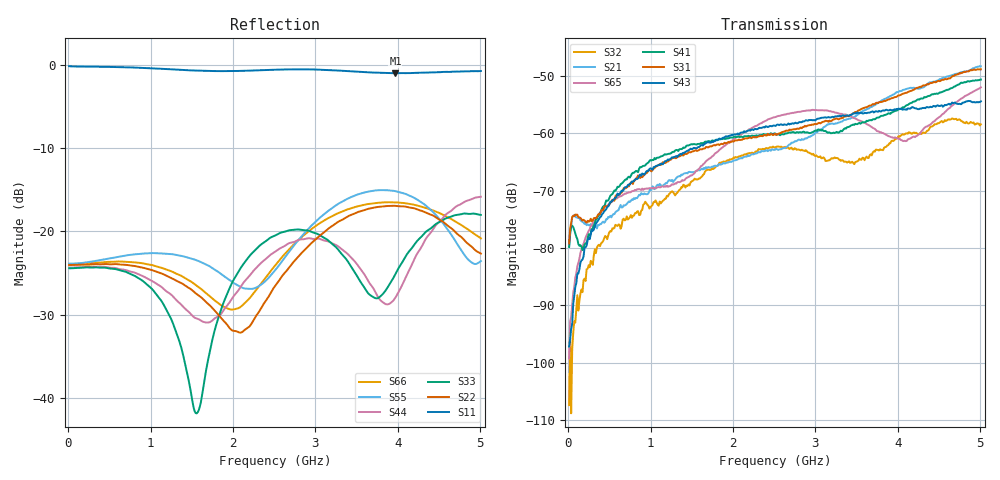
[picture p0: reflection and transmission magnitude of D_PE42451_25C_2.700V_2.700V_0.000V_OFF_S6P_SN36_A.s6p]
! Device ID: PE42451
! Serial: 36
! Insertion: A
! Temp: 25C
! VDD: 2.700
! Control_Hi: 100.000
! Control_Lo: 0.000
! Logic State: OFF
! Port 1: RFC
! Port 2: RF1
! Port 3: RF2
! Port 4: RF3
! Port 5: RF4
! Port 6: RF5
! V1 = 0.00
! V2 = 2.70
! V3 = 2.70
! V4 = 0.00
! IDD: 1.083360e-05
#  Hz  S  RI  R  50
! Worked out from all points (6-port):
!   401 points, 10 MHz to 5.01 GHz, reference 50 ohm
!   strongest paths, dB at 10 MHz, 1.26 GHz, 2.51 GHz, 3.76 GHz, 5.01 GHz:
!     S43: -97.2, -64.2, -58.7, -56.2, -54.4
!     S31: -79.2, -64.4, -60.1, -54.7, -48.8
!     S41: -79.8, -63.3, -60.0, -57.2, -50.6
!     S65: -99.3, -68.9, -57.2, -59.7, -52.0
!     S21: -79.8, -68.1, -62.9, -54.7, -48.3
!     S32: -107.4, -70.1, -62.5, -62.9, -58.4
!   lowest |S11| = -1.0 dB at 3.973 GHz (marker M1), VSWR 18.06, Z = 3 - j14.5 ohm
!   |S11| at or under -10 dB: nowhere
